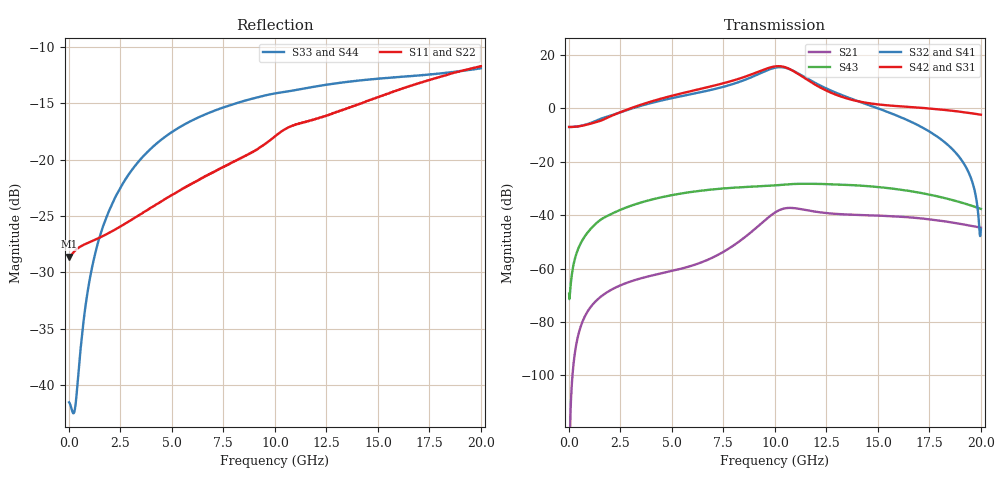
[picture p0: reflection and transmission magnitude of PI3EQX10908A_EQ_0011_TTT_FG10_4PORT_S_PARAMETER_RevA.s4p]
! NPort=4 DATA=2000 NOISE=0 GROUPDELAY=0 COMPLEX_DATAFORMAT=POLAR
! NumOfBlock=1 NumOfParam=0
! .MODEL Smodel S TSTONEFILE=PI3EQX10908A_EQ_0011_TTT_FG10_4PORT_S_PARAMETER_RevA.s4p TYPE=S
!  -- The above .MODEL line can be used for the S element in the netlist.
! The s parameter is extracted from the linear redriver, it is not bi-directional; only s(4,1)s(4,2) and s(3,1)s(3,2)
! should be the insertion loss
!Port definition:
!Port1 = input+
!Port2 = input-
!Port3 = output+
!Port4 = output-
# Hz S MA R  50
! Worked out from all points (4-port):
!   2000 points, 10 MHz to 20 GHz, reference 50 ohm
!   strongest paths, dB at 10 MHz, 5.01 GHz, 10.01 GHz, 15.01 GHz, 20 GHz:
!     S42: -6.9, 4.8, 15.7, 1.5, -2.3
!     S31: -6.9, 4.8, 15.7, 1.5, -2.3
!     S32: -6.9, 3.9, 15.3, 0.0, -45.2
!     S41: -6.9, 3.9, 15.3, 0.0, -44.7
!     S43: -69.4, -32.4, -28.8, -29.4, -37.6
!     S21: -127.3, -60.8, -38.9, -40.1, -44.6
!   lowest |S11| = -28.6 dB at 10 MHz (marker M1), VSWR 1.08, Z = 46.4 - j0.024 ohm
!   |S11| at or under -10 dB: start of sweep to end of sweep
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1e7  0.03701 -179.6  4.328e-07 13.6  0 0.0  0 0.0
     4.328e-07 13.6  0.03701 -179.6  0 0.0  0 0.0
     0.4502 -0.0  0.4502 180.0  0.008374 26.0  0.00034 -27.1
     0.4502 180.0  0.4502 -0.0  0.00034 -27.1  0.008374 26.0
8e9  0.09783 -116.6  0.002735 135.1  1.193e-06 48.7  4.811e-07 132.4
     0.002735 135.2  0.09787 -116.6  4.812e-07 132.4  1.193e-06 48.7
     3.358 -58.1  2.897 115.7  0.1763 1.7  0.03283 3.0
     2.898 115.7  3.358 -58.1  0.03283 3.0  0.1763 1.7
9.73e9  0.1209 -110.6  0.009423 117.4  4.368e-06 6.7  2.755e-06 120.8
        0.009426 117.5  0.121 -110.6  2.756e-06 120.8  4.369e-06 6.7
        5.791 -110.7  5.375 64.0  0.1943 -11.0  0.03567 -13.7
        5.376 64.0  5.791 -110.7  0.03567 -13.7  0.1943 -11.0
1.06e10  0.1379 -111.3  0.01367 78.5  5.616e-06 -27.6  6.165e-06 82.6
         0.01367 78.5  0.138 -111.3  6.167e-06 82.6  5.617e-06 -27.6
         5.722 -159.7  5.641 13.2  0.2004 -16.7  0.03798 -22.7
         5.641 13.2  5.723 -159.7  0.03798 -22.7  0.2004 -16.7
1.155e10  0.1474 -112.7  0.01244 46.0  5.417e-06 -35.2  8.898e-06 45.0
          0.01243 46.0  0.1475 -112.7  8.901e-06 45.0  5.417e-06 -35.2
          3.473 162.5  3.659 -29.3  0.2076 -21.8  0.03887 -35.0
          3.658 -29.3  3.473 162.5  0.03887 -35.0  0.2076 -21.8
1.369e10  0.171 -111.3  0.01026 15.7  1.41e-05 -39.2  1.748e-05 -4.6
          0.01025 15.8  0.1711 -111.3  1.748e-05 -4.6  1.409e-05 -39.2
          1.467 137.7  1.531 -75.8  0.2222 -33.0  0.0368 -61.2
          1.53 -75.8  1.467 137.8  0.0368 -61.2  0.2222 -33.0
2e10  0.2595 -114.1  0.005867 -45.2  9.151e-05 -147.8  7.233e-05 -137.1
      0.005859 -44.9  0.2596 -114.1  7.234e-05 -137.1  9.15e-05 -147.8
      0.7636 61.2  0.005473 -60.8  0.2539 -52.2  0.01317 -136.8
      0.005833 -67.9  0.7643 61.2  0.01317 -136.8  0.2539 -52.2
